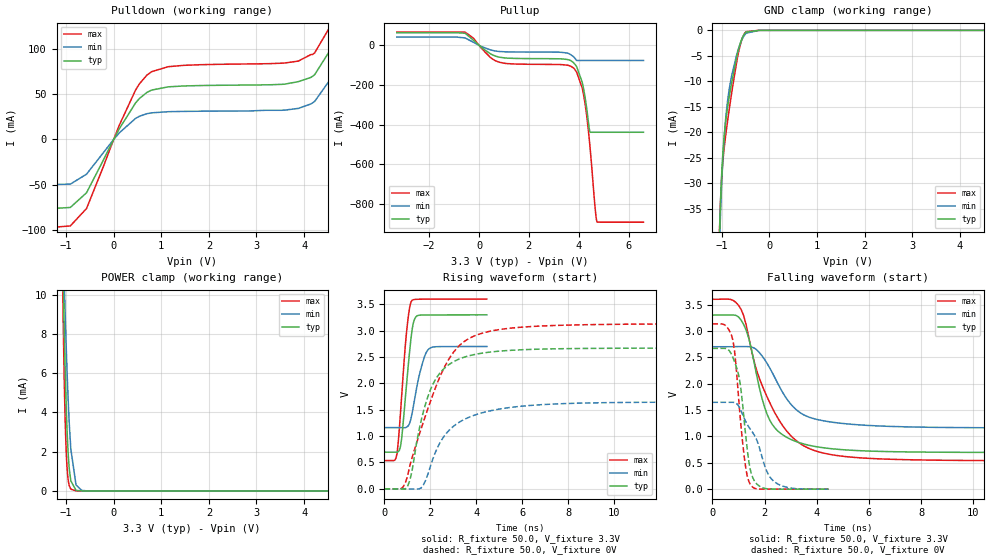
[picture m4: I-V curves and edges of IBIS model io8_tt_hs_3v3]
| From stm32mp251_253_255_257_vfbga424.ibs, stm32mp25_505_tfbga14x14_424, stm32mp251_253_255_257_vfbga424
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[Model]   io8_tt_hs_3v3
Model_type I/O
Polarity   Non-Inverting
Enable   Active-Low
| CAP_THRESHOLD on pad IOTT is "UDTCAPC" :
| Rising=30.0% of vddiov33m   Falling=70.0% of vddiov33m
| C_comp min and max val. don't necessarily correlate with the min and max pvt
| but are the smallest and greatest pad capacitance found.
| var   typ   min   max
C_comp   1.24002pF  995.40444fF  2.17633pF
|C_comp_pullup   730.17000fF  473.44500fF  1.67078pF
|C_comp_pulldown   509.85000fF  521.95944fF  505.54500fF
Vinl = 810.0mV
Vinh = 2.52V
Vmeas = 1.65V   | Reference voltage for timing measurements
Cref  = 50.0pF   | Timing specification test load capacitance value
Rref  = 100.0MOhm   | Timing specification test load resistance value
Vref  = 1.65V   | Timing specification test load voltage
[Model Spec]
| TIME_THRESHOLD on pin ZIV08M is "CMOS" :
| Rising=50.0% of vddv08m   Falling=50.0% of vddv08m
Vinl 1.08570V 868.70000mV 1.21270V
Vinh 1.55630V 1.26330V 1.71030V
| variable   typ   min   max
[Temperature Range] 25.0 125.0 -40.0
| variable   typ   min   max
[Voltage Range] 3.3V 2.7V 3.6V
| variable   typ   min   max
[POWER Clamp Reference] 3.3V 2.7V 3.6V
| variable   typ   min   max
[GND Clamp Reference] 0V 0V 0V
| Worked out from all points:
|   slope of the pulldown table from 0 to 0.495 V, typ, clamps not added: 11.6 ohm
|   slope of the pullup table from 0 to 0.495 V, typ, clamps not added: 10.9 ohm
|   GND clamp passes 1 mA (typ) near -0.55 V on its own axis
|   POWER clamp passes 1 mA (typ) near -0.93 V on its own axis
|   rising waveform, R_fixture 50.0, V_fixture 3.3V: 20-80 % time 329ps typ, 443ps min, 316ps max; typ from 0.695 V to 3.3 V
|   falling waveform, R_fixture 50.0, V_fixture 3.3V: 20-80 % time 876ps typ, 1.22ns min, 1.43ns max; typ from 3.3 V to 0.695 V
|   rising waveform, R_fixture 50.0, V_fixture 0V: 20-80 % time 1.04ns typ, 1.55ns min, 1.64ns max; typ from 0 V to 2.67 V
|   falling waveform, R_fixture 50.0, V_fixture 0V: 20-80 % time 379ps typ, 850ps min, 346ps max; typ from 2.67 V to 0 V
[POWER Clamp]
-3.3V     1.352A     318.4mA    1.997A
-1.07V    12.07mA    13.62mA    10.38mA
-1.06V    10.79mA    12.67mA    8.742mA
-1.05V    9.57mA     11.75mA    7.25mA
-1.03V    7.34mA     9.996mA    4.745mA
-1V       4.587mA    7.593mA    2.212mA
-980mV    3.182mA    6.169mA    1.235mA
-950mV    1.703mA    4.334mA    479uA
-900mV    514.7uA    2.139mA    90.77uA
-790mV    28.73uA    299.9uA    2.711uA
-670mV    1.278uA    27.54uA    387.5nA
6.6V      0A         0A         0A
[GND Clamp]
-3.3V     -3.764A    -3.734A    -3.781A
-1.05V    -39.76mA   -42.44mA   -39.2mA
-1.04V    -36.65mA   -39.24mA   -36.3mA
-1.03V    -33.91mA   -36.36mA   -33.82mA
-1V       -27.43mA   -29.21mA   -28.35mA
-970mV    -22.87mA   -23.78mA   -24.78mA
-920mV    -17.9mA    -17.36mA   -20.6mA
-860mV    -13.88mA   -12.47mA   -16.46mA
-790mV    -10.04mA   -8.727mA   -11.99mA
-650mV    -3.744mA   -3.565mA   -4.327mA
-490mV    -324.2uA   -555.2uA   -259.7uA
6.6V      204.7nA    4.775uA    218.9nA
| variable   typ   min   max
[Pullup Reference] 3.3V 2.7V 3.6V
| variable   typ   min   max
[Pulldown Reference] 0V 0V 0V
[Pullup]
-3.3V     63.52mA    41.46mA    66.64mA
-560mV    60.73mA    37.23mA    66.64mA
800mV     -59.67mA   -31.11mA   -85.07mA
3.3V      -68.5mA    -35.37mA   -97.42mA
3.79V     -87.42mA   -57.41mA   -114.2mA
3.92V     -108.3mA   -76.54mA   -136.5mA
4.14V     -186.3mA   -76.54mA   -215.1mA
4.25V     -258.3mA   -76.54mA   -290.8mA
4.45V     -435.4mA   -76.54mA   -508.5mA
4.65V     -438.9mA   -76.54mA   -809mA
4.73V     -438.9mA   -76.54mA   -889.8mA
6.6V      -438.9mA   -76.54mA   -892.6mA
[Pulldown]
-3.3V     -76.42mA   -49.85mA   -97.23mA
-910mV    -75.34mA   -49.51mA   -95.8mA
-570mV    -59.08mA   -38.48mA   -76.52mA
120mV     12mA       7.376mA    15.98mA
460mV     40.46mA    23.32mA    54.73mA
800mV     54.75mA    29.51mA    75.15mA
1.48V     59.3mA     31.12mA    82.16mA
3.88V     64.11mA    34.44mA    86.87mA
4.22V     71.69mA    42.05mA    95.8mA
4.56V     99.99mA    67.27mA    126.4mA
4.9V      185.2mA    140.4mA    220.4mA
6.6V      1.448A     1.604A     1.428A
[Ramp]
dV/dt_r 1.60187V/1.03331ns 987.9854mV/1.54471ns 1.87964V/1.64146ns
dV/dt_f 1.5628V/872.07056ps 923.4803mV/1.22207ns 1.83839V/1.42413ns
R_load = 50.0
| Removed startup time: 0s 0s 0s  .
| Removed end time: 4.45ns.
[Rising Waveform]
R_fixture   = 50.0
V_fixture   = 3.3V
V_fixture_min = 2.7V
V_fixture_max = 3.6V
0s        695.3mV    1.161V     536mV
550ps     693.1mV    1.161V     675.9mV
750ps     957.2mV    1.161V     1.771V
950ps     1.923V     1.167V     2.922V
1.1ns     2.632V     1.25V      3.453V
1.2ns     3.011V     1.426V     3.575V
1.35ns    3.252V     1.794V     3.594V
1.55ns    3.295V     2.218V     3.597V
1.95ns    3.298V     2.659V     3.599V
4.45ns    3.3V       2.7V       3.6V
| Removed startup time: 0s 0s 0s  .
| Removed end time: 24.9ns.
[Falling Waveform]
R_fixture   = 50.0
V_fixture   = 3.3V
V_fixture_min = 2.7V
V_fixture_max = 3.6V
0s        3.3V       2.7V       3.6V
800ps     3.303V     2.7V       3.577V
1.2ns     3.121V     2.702V     3.289V
1.4ns     2.853V     2.701V     2.869V
1.7ns     2.154V     2.642V     2.245V
2ns       1.557V     2.46V      1.858V
2.4ns     1.159V     2.109V     1.441V
3.2ns     904.6mV    1.513V     926.4mV
4.2ns     788.9mV    1.302V     690.8mV
24.9ns    695.3mV    1.161V     536mV
| Removed startup time: 0s 0s 0s  .
| Removed end time: 24.9ns.
[Rising Waveform]
R_fixture   = 50.0
V_fixture   = 0V
V_fixture_min = 0V
V_fixture_max = 0V
0s        255.5nV    1.557uV    317.8nV
700ps     -5.142mV   -90.28uV   -1.384mV
1ns       42.98mV    -2.187mV   234.1mV
1.2ns     339.8mV    -4.043mV   590.1mV
1.7ns     1.476V     77.5mV     1.277V
2.3ns     2.131V     776.9mV    2.009V
3.2ns     2.454V     1.249V     2.693V
4.3ns     2.577V     1.448V     2.959V
8.7ns     2.663V     1.627V     3.113V
24.9ns    2.67V      1.647V     3.133V
| Removed startup time: 0s 0s 0s  .
| Removed end time: 4.45ns.
[Falling Waveform]
R_fixture   = 50.0
V_fixture   = 0V
V_fixture_min = 0V
V_fixture_max = 0V
0s        2.67V      1.647V     3.133V
750ps     2.541V     1.647V     2.894V
850ps     2.414V     1.643V     2.619V
1.05ns    2.05V      1.537V     1.453V
1.25ns    1.149V     1.312V     503mV
1.45ns    378.9mV    1.141V     94.94mV
1.75ns    77.71mV    868.7mV    3.733mV
2.1ns     7.169mV    323.8mV    1.229mV
2.4ns     1.089mV    132.1mV    825.7uV
4.45ns    142.2uV    288.6uV    170.4uV
